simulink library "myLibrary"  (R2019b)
settings: Solver=VariableStepAuto  StartTime=0.0  StopTime=10.0  RelTol=1e-3
undefined symbols (not defined in the file or in its folder): batt_delay, Calculation, cap_1ph, cap_3ph, Complex, Current, Dynamic, EV, ev_charger, EV_ID, ev_num, gcbh, Iabc, Load, max_charge_1ph, max_charge_3ph, max_disch_1ph, max_disch_3ph, MV_LV_transf, myLibrary, phase, Phase, Phasor, rated_1ph, rated_3ph, Single, SoC_init, SPDL, sps_rtmsupport, Tr_capacity, Tstep, Vabc, Vnom, yes
libraries: powerlib x163, $bdroot x13, spsVIMeasurementModel x3, simulink x2, powerlib_meascontrol x1
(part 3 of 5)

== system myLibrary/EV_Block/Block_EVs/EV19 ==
  Breaker : powerlib/Elements/Breaker  InitialState=1  SwitchingTimes=0  External=off  BreakerResistance=0.01  SnubberResistance=1e3  SnubberCapacitance=inf  Measurements=None  MoreParameters=on  NoBreakLoop=off
  Controlled Current Source : powerlib/Electrical Sources/Controlled Current Source  Initialize=on  Source_Type=AC  Amplitude=0  Phase=0  Frequency=50  Measurements=None
  Current Calculation : Subsystem
  Gain : Gain  Gain=sqrt(2)
  Initialization : Subsystem
  Snubber4 : powerlib/Elements/Series RLC Branch  LConnTagsString=__new0  RConnTagsString=__new0  BranchType=R  Resistance=1e6  Inductance=1e-3  SetiL0=off  InitialCurrent=0  Capacitance=1e-6  Setx0=off  InitialVoltage=0  Measurements=None
  Step : Step  Time=0.001  Before=-1  SampleTime=0
  Switch : Switch  Criteria=u2 > Threshold
  Voltage Measurement : powerlib/Measurements/Voltage Measurement  PhasorSimulation=off  OutputType=Complex  PSBequivalent=0
  Phase : PMIOPort  Side=Left
  Neutral : PMIOPort  Port=2  Side=Left
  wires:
  Gain/1 -> Switch/3
  Step/1 -> Switch/2
  Initialization/1(Out1) -> Gain/1
  [Vm_c] -> Switch/1
  [Icontrol] -> Controlled Current Source/1
  Current Calculation/1(Isignal) -> [Icontrol]
  Switch/1 -> Current Calculation/1(Vp)
  Voltage Measurement/1 -> [Vm_c]
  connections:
  Snubber4/LConn1 -- Breaker/LConn1
  Phase/RConn1 -- Voltage Measurement/LConn1 -- Breaker/RConn1 -- Controlled Current Source/LConn1
  Neutral/RConn1 -- Controlled Current Source/RConn1 -- Snubber4/RConn1 -- Voltage Measurement/LConn2

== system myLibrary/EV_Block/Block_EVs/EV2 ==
  Breaker : powerlib/Elements/Breaker  InitialState=1  SwitchingTimes=0  External=off  BreakerResistance=0.01  SnubberResistance=1e3  SnubberCapacitance=inf  Measurements=None  MoreParameters=on  NoBreakLoop=off
  Controlled Current Source : powerlib/Electrical Sources/Controlled Current Source  Initialize=on  Source_Type=AC  Amplitude=0  Phase=0  Frequency=50  Measurements=None
  Current Calculation : Subsystem
  Gain : Gain  Gain=sqrt(2)
  Initialization : Subsystem
  Snubber4 : powerlib/Elements/Series RLC Branch  LConnTagsString=__new0  RConnTagsString=__new0  BranchType=R  Resistance=1e6  Inductance=1e-3  SetiL0=off  InitialCurrent=0  Capacitance=1e-6  Setx0=off  InitialVoltage=0  Measurements=None
  Step : Step  Time=0.001  Before=-1  SampleTime=0
  Switch : Switch  Criteria=u2 > Threshold
  Voltage Measurement : powerlib/Measurements/Voltage Measurement  PhasorSimulation=off  OutputType=Complex  PSBequivalent=0
  Phase : PMIOPort  Side=Left
  Neutral : PMIOPort  Port=2  Side=Left
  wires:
  Gain/1 -> Switch/3
  Step/1 -> Switch/2
  Initialization/1(Out1) -> Gain/1
  [Vm_c] -> Switch/1
  [Icontrol] -> Controlled Current Source/1
  Current Calculation/1(Isignal) -> [Icontrol]
  Switch/1 -> Current Calculation/1(Vp)
  Voltage Measurement/1 -> [Vm_c]
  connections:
  Snubber4/LConn1 -- Breaker/LConn1
  Phase/RConn1 -- Voltage Measurement/LConn1 -- Breaker/RConn1 -- Controlled Current Source/LConn1
  Neutral/RConn1 -- Controlled Current Source/RConn1 -- Snubber4/RConn1 -- Voltage Measurement/LConn2

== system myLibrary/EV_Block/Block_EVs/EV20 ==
  Breaker : powerlib/Elements/Breaker  InitialState=1  SwitchingTimes=0  External=off  BreakerResistance=0.01  SnubberResistance=1e3  SnubberCapacitance=inf  Measurements=None  MoreParameters=on  NoBreakLoop=off
  Controlled Current Source : powerlib/Electrical Sources/Controlled Current Source  Initialize=on  Source_Type=AC  Amplitude=0  Phase=0  Frequency=50  Measurements=None
  Current Calculation : Subsystem
  Gain : Gain  Gain=sqrt(2)
  Initialization : Subsystem
  Snubber4 : powerlib/Elements/Series RLC Branch  LConnTagsString=__new0  RConnTagsString=__new0  BranchType=R  Resistance=1e6  Inductance=1e-3  SetiL0=off  InitialCurrent=0  Capacitance=1e-6  Setx0=off  InitialVoltage=0  Measurements=None
  Step : Step  Time=0.001  Before=-1  SampleTime=0
  Switch : Switch  Criteria=u2 > Threshold
  Voltage Measurement : powerlib/Measurements/Voltage Measurement  PhasorSimulation=off  OutputType=Complex  PSBequivalent=0
  Phase : PMIOPort  Side=Left
  Neutral : PMIOPort  Port=2  Side=Left
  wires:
  Gain/1 -> Switch/3
  Step/1 -> Switch/2
  Initialization/1(Out1) -> Gain/1
  [Vm_c] -> Switch/1
  [Icontrol] -> Controlled Current Source/1
  Current Calculation/1(Isignal) -> [Icontrol]
  Switch/1 -> Current Calculation/1(Vp)
  Voltage Measurement/1 -> [Vm_c]
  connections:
  Snubber4/LConn1 -- Breaker/LConn1
  Phase/RConn1 -- Voltage Measurement/LConn1 -- Breaker/RConn1 -- Controlled Current Source/LConn1
  Neutral/RConn1 -- Controlled Current Source/RConn1 -- Snubber4/RConn1 -- Voltage Measurement/LConn2

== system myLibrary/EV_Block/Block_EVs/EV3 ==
  Breaker : powerlib/Elements/Breaker  InitialState=1  SwitchingTimes=0  External=off  BreakerResistance=0.01  SnubberResistance=1e3  SnubberCapacitance=inf  Measurements=None  MoreParameters=on  NoBreakLoop=off
  Controlled Current Source : powerlib/Electrical Sources/Controlled Current Source  Initialize=on  Source_Type=AC  Amplitude=0  Phase=0  Frequency=50  Measurements=None
  Current Calculation : Subsystem
  Gain : Gain  Gain=sqrt(2)
  Initialization : Subsystem
  Snubber4 : powerlib/Elements/Series RLC Branch  LConnTagsString=__new0  RConnTagsString=__new0  BranchType=R  Resistance=1e6  Inductance=1e-3  SetiL0=off  InitialCurrent=0  Capacitance=1e-6  Setx0=off  InitialVoltage=0  Measurements=None
  Step : Step  Time=0.001  Before=-1  SampleTime=0
  Switch : Switch  Criteria=u2 > Threshold
  Voltage Measurement : powerlib/Measurements/Voltage Measurement  PhasorSimulation=off  OutputType=Complex  PSBequivalent=0
  Phase : PMIOPort  Side=Left
  Neutral : PMIOPort  Port=2  Side=Left
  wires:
  Gain/1 -> Switch/3
  Step/1 -> Switch/2
  Initialization/1(Out1) -> Gain/1
  [Vm_c] -> Switch/1
  [Icontrol] -> Controlled Current Source/1
  Current Calculation/1(Isignal) -> [Icontrol]
  Switch/1 -> Current Calculation/1(Vp)
  Voltage Measurement/1 -> [Vm_c]
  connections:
  Snubber4/LConn1 -- Breaker/LConn1
  Phase/RConn1 -- Voltage Measurement/LConn1 -- Breaker/RConn1 -- Controlled Current Source/LConn1
  Neutral/RConn1 -- Controlled Current Source/RConn1 -- Snubber4/RConn1 -- Voltage Measurement/LConn2

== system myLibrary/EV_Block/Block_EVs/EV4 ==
  Breaker : powerlib/Elements/Breaker  InitialState=1  SwitchingTimes=0  External=off  BreakerResistance=0.01  SnubberResistance=1e3  SnubberCapacitance=inf  Measurements=None  MoreParameters=on  NoBreakLoop=off
  Controlled Current Source : powerlib/Electrical Sources/Controlled Current Source  Initialize=on  Source_Type=AC  Amplitude=0  Phase=0  Frequency=50  Measurements=None
  Current Calculation : Subsystem
  Gain : Gain  Gain=sqrt(2)
  Initialization : Subsystem
  Snubber4 : powerlib/Elements/Series RLC Branch  LConnTagsString=__new0  RConnTagsString=__new0  BranchType=R  Resistance=1e6  Inductance=1e-3  SetiL0=off  InitialCurrent=0  Capacitance=1e-6  Setx0=off  InitialVoltage=0  Measurements=None
  Step : Step  Time=0.001  Before=-1  SampleTime=0
  Switch : Switch  Criteria=u2 > Threshold
  Voltage Measurement : powerlib/Measurements/Voltage Measurement  PhasorSimulation=off  OutputType=Complex  PSBequivalent=0
  Phase : PMIOPort  Side=Left
  Neutral : PMIOPort  Port=2  Side=Left
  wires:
  Gain/1 -> Switch/3
  Step/1 -> Switch/2
  Initialization/1(Out1) -> Gain/1
  [Vm_c] -> Switch/1
  [Icontrol] -> Controlled Current Source/1
  Current Calculation/1(Isignal) -> [Icontrol]
  Switch/1 -> Current Calculation/1(Vp)
  Voltage Measurement/1 -> [Vm_c]
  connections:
  Snubber4/LConn1 -- Breaker/LConn1
  Phase/RConn1 -- Voltage Measurement/LConn1 -- Breaker/RConn1 -- Controlled Current Source/LConn1
  Neutral/RConn1 -- Controlled Current Source/RConn1 -- Snubber4/RConn1 -- Voltage Measurement/LConn2

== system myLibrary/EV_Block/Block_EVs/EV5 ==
  Breaker : powerlib/Elements/Breaker  InitialState=1  SwitchingTimes=0  External=off  BreakerResistance=0.01  SnubberResistance=1e3  SnubberCapacitance=inf  Measurements=None  MoreParameters=on  NoBreakLoop=off
  Controlled Current Source : powerlib/Electrical Sources/Controlled Current Source  Initialize=on  Source_Type=AC  Amplitude=0  Phase=0  Frequency=50  Measurements=None
  Current Calculation : Subsystem
  Gain : Gain  Gain=sqrt(2)
  Initialization : Subsystem
  Snubber4 : powerlib/Elements/Series RLC Branch  LConnTagsString=__new0  RConnTagsString=__new0  BranchType=R  Resistance=1e6  Inductance=1e-3  SetiL0=off  InitialCurrent=0  Capacitance=1e-6  Setx0=off  InitialVoltage=0  Measurements=None
  Step : Step  Time=0.001  Before=-1  SampleTime=0
  Switch : Switch  Criteria=u2 > Threshold
  Voltage Measurement : powerlib/Measurements/Voltage Measurement  PhasorSimulation=off  OutputType=Complex  PSBequivalent=0
  Phase : PMIOPort  Side=Left
  Neutral : PMIOPort  Port=2  Side=Left
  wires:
  Gain/1 -> Switch/3
  Step/1 -> Switch/2
  Initialization/1(Out1) -> Gain/1
  [Vm_c] -> Switch/1
  [Icontrol] -> Controlled Current Source/1
  Current Calculation/1(Isignal) -> [Icontrol]
  Switch/1 -> Current Calculation/1(Vp)
  Voltage Measurement/1 -> [Vm_c]
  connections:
  Snubber4/LConn1 -- Breaker/LConn1
  Phase/RConn1 -- Voltage Measurement/LConn1 -- Breaker/RConn1 -- Controlled Current Source/LConn1
  Neutral/RConn1 -- Controlled Current Source/RConn1 -- Snubber4/RConn1 -- Voltage Measurement/LConn2

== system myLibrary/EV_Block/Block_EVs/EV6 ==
  Breaker : powerlib/Elements/Breaker  InitialState=1  SwitchingTimes=0  External=off  BreakerResistance=0.01  SnubberResistance=1e3  SnubberCapacitance=inf  Measurements=None  MoreParameters=on  NoBreakLoop=off
  Controlled Current Source : powerlib/Electrical Sources/Controlled Current Source  Initialize=on  Source_Type=AC  Amplitude=0  Phase=0  Frequency=50  Measurements=None
  Current Calculation : Subsystem
  Gain : Gain  Gain=sqrt(2)
  Initialization : Subsystem
  Snubber4 : powerlib/Elements/Series RLC Branch  LConnTagsString=__new0  RConnTagsString=__new0  BranchType=R  Resistance=1e6  Inductance=1e-3  SetiL0=off  InitialCurrent=0  Capacitance=1e-6  Setx0=off  InitialVoltage=0  Measurements=None
  Step : Step  Time=0.001  Before=-1  SampleTime=0
  Switch : Switch  Criteria=u2 > Threshold
  Voltage Measurement : powerlib/Measurements/Voltage Measurement  PhasorSimulation=off  OutputType=Complex  PSBequivalent=0
  Phase : PMIOPort  Side=Left
  Neutral : PMIOPort  Port=2  Side=Left
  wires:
  Gain/1 -> Switch/3
  Step/1 -> Switch/2
  Initialization/1(Out1) -> Gain/1
  [Vm_c] -> Switch/1
  [Icontrol] -> Controlled Current Source/1
  Current Calculation/1(Isignal) -> [Icontrol]
  Switch/1 -> Current Calculation/1(Vp)
  Voltage Measurement/1 -> [Vm_c]
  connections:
  Snubber4/LConn1 -- Breaker/LConn1
  Phase/RConn1 -- Voltage Measurement/LConn1 -- Breaker/RConn1 -- Controlled Current Source/LConn1
  Neutral/RConn1 -- Controlled Current Source/RConn1 -- Snubber4/RConn1 -- Voltage Measurement/LConn2

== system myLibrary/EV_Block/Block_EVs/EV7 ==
  Breaker : powerlib/Elements/Breaker  InitialState=1  SwitchingTimes=0  External=off  BreakerResistance=0.01  SnubberResistance=1e3  SnubberCapacitance=inf  Measurements=None  MoreParameters=on  NoBreakLoop=off
  Controlled Current Source : powerlib/Electrical Sources/Controlled Current Source  Initialize=on  Source_Type=AC  Amplitude=0  Phase=0  Frequency=50  Measurements=None
  Current Calculation : Subsystem
  Gain : Gain  Gain=sqrt(2)
  Initialization : Subsystem
  Snubber4 : powerlib/Elements/Series RLC Branch  LConnTagsString=__new0  RConnTagsString=__new0  BranchType=R  Resistance=1e6  Inductance=1e-3  SetiL0=off  InitialCurrent=0  Capacitance=1e-6  Setx0=off  InitialVoltage=0  Measurements=None
  Step : Step  Time=0.001  Before=-1  SampleTime=0
  Switch : Switch  Criteria=u2 > Threshold
  Voltage Measurement : powerlib/Measurements/Voltage Measurement  PhasorSimulation=off  OutputType=Complex  PSBequivalent=0
  Phase : PMIOPort  Side=Left
  Neutral : PMIOPort  Port=2  Side=Left
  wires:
  Gain/1 -> Switch/3
  Step/1 -> Switch/2
  Initialization/1(Out1) -> Gain/1
  [Vm_c] -> Switch/1
  [Icontrol] -> Controlled Current Source/1
  Current Calculation/1(Isignal) -> [Icontrol]
  Switch/1 -> Current Calculation/1(Vp)
  Voltage Measurement/1 -> [Vm_c]
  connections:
  Snubber4/LConn1 -- Breaker/LConn1
  Phase/RConn1 -- Voltage Measurement/LConn1 -- Breaker/RConn1 -- Controlled Current Source/LConn1
  Neutral/RConn1 -- Controlled Current Source/RConn1 -- Snubber4/RConn1 -- Voltage Measurement/LConn2

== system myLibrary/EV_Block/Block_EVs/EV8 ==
  Breaker : powerlib/Elements/Breaker  InitialState=1  SwitchingTimes=0  External=off  BreakerResistance=0.01  SnubberResistance=1e3  SnubberCapacitance=inf  Measurements=None  MoreParameters=on  NoBreakLoop=off
  Controlled Current Source : powerlib/Electrical Sources/Controlled Current Source  Initialize=on  Source_Type=AC  Amplitude=0  Phase=0  Frequency=50  Measurements=None
  Current Calculation : Subsystem
  Gain : Gain  Gain=sqrt(2)
  Initialization : Subsystem
  Snubber4 : powerlib/Elements/Series RLC Branch  LConnTagsString=__new0  RConnTagsString=__new0  BranchType=R  Resistance=1e6  Inductance=1e-3  SetiL0=off  InitialCurrent=0  Capacitance=1e-6  Setx0=off  InitialVoltage=0  Measurements=None
  Step : Step  Time=0.001  Before=-1  SampleTime=0
  Switch : Switch  Criteria=u2 > Threshold
  Voltage Measurement : powerlib/Measurements/Voltage Measurement  PhasorSimulation=off  OutputType=Complex  PSBequivalent=0
  Phase : PMIOPort  Side=Left
  Neutral : PMIOPort  Port=2  Side=Left
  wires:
  Gain/1 -> Switch/3
  Step/1 -> Switch/2
  Initialization/1(Out1) -> Gain/1
  [Vm_c] -> Switch/1
  [Icontrol] -> Controlled Current Source/1
  Current Calculation/1(Isignal) -> [Icontrol]
  Switch/1 -> Current Calculation/1(Vp)
  Voltage Measurement/1 -> [Vm_c]
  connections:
  Snubber4/LConn1 -- Breaker/LConn1
  Phase/RConn1 -- Voltage Measurement/LConn1 -- Breaker/RConn1 -- Controlled Current Source/LConn1
  Neutral/RConn1 -- Controlled Current Source/RConn1 -- Snubber4/RConn1 -- Voltage Measurement/LConn2

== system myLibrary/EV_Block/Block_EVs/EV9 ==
  Breaker : powerlib/Elements/Breaker  InitialState=1  SwitchingTimes=0  External=off  BreakerResistance=0.01  SnubberResistance=1e3  SnubberCapacitance=inf  Measurements=None  MoreParameters=on  NoBreakLoop=off
  Controlled Current Source : powerlib/Electrical Sources/Controlled Current Source  Initialize=on  Source_Type=AC  Amplitude=0  Phase=0  Frequency=50  Measurements=None
  Current Calculation : Subsystem
  Gain : Gain  Gain=sqrt(2)
  Initialization : Subsystem
  Snubber4 : powerlib/Elements/Series RLC Branch  LConnTagsString=__new0  RConnTagsString=__new0  BranchType=R  Resistance=1e6  Inductance=1e-3  SetiL0=off  InitialCurrent=0  Capacitance=1e-6  Setx0=off  InitialVoltage=0  Measurements=None
  Step : Step  Time=0.001  Before=-1  SampleTime=0
  Switch : Switch  Criteria=u2 > Threshold
  Voltage Measurement : powerlib/Measurements/Voltage Measurement  PhasorSimulation=off  OutputType=Complex  PSBequivalent=0
  Phase : PMIOPort  Side=Left
  Neutral : PMIOPort  Port=2  Side=Left
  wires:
  Gain/1 -> Switch/3
  Step/1 -> Switch/2
  Initialization/1(Out1) -> Gain/1
  [Vm_c] -> Switch/1
  [Icontrol] -> Controlled Current Source/1
  Current Calculation/1(Isignal) -> [Icontrol]
  Switch/1 -> Current Calculation/1(Vp)
  Voltage Measurement/1 -> [Vm_c]
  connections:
  Snubber4/LConn1 -- Breaker/LConn1
  Phase/RConn1 -- Voltage Measurement/LConn1 -- Breaker/RConn1 -- Controlled Current Source/LConn1
  Neutral/RConn1 -- Controlled Current Source/RConn1 -- Snubber4/RConn1 -- Voltage Measurement/LConn2

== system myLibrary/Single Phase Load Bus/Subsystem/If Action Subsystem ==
  Action Port : ActionPort
  Constant : Constant
  Out1 : Outport  VectorParamsAs1DForOutWhenUnconnected=off
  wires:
  Constant/1 -> Out1/1

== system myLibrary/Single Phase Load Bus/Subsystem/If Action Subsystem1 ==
  Action Port : ActionPort
  Constant : Constant
  Out1 : Outport  VectorParamsAs1DForOutWhenUnconnected=off
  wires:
  Constant/1 -> Out1/1

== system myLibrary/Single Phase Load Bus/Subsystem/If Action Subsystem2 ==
  Action Port : ActionPort
  Constant : Constant
  Out1 : Outport  VectorParamsAs1DForOutWhenUnconnected=off
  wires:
  Constant/1 -> Out1/1

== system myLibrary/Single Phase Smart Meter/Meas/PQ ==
  V : Inport
  I : Inport  Port=2
  Complex to Real-Imag : ComplexToRealImag
  Constant : Constant  Value=2
  Divide : Product  Inputs=*/
  Math Function : Math  Operator=conj
  Product : Product
  P : Outport  VectorParamsAs1DForOutWhenUnconnected=off
  Q : Outport  Port=2  VectorParamsAs1DForOutWhenUnconnected=off
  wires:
  I/1 -> Math Function/1
  V/1 -> Product/1
  Math Function/1 -> Product/2
  Product/1 -> Divide/1
  Constant/1 -> Divide/2
  Divide/1 -> Complex to Real-Imag/1
  Complex to Real-Imag/1 -> P/1
  Complex to Real-Imag/2 -> Q/1

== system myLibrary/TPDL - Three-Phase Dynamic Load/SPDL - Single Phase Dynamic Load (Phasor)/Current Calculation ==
  Vp : Inport
  Demux : Demux  Outputs=6
  Divide : Product  Inputs=*/
  From Workspace : FromWorkspace  VariableName=Load_Profile  SampleTime=0  OutputAfterFinalValue=Holding final value
  Gain : Gain  Gain=2
  Math Function : Math  Operator=conj
  Real-Imag to Complex : RealImagToComplex
  Isignal : Outport  VectorParamsAs1DForOutWhenUnconnected=off
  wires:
  Vp/1 -> Divide/2
  Gain/1 -> Divide/1
  Divide/1 -> Math Function/1
  Math Function/1 -> Isignal/1
  From Workspace/1 -> Demux/1
  Demux/1 -> Real-Imag to Complex/1
  Demux/2 -> Real-Imag to Complex/2
  Real-Imag to Complex/1 -> Gain/1

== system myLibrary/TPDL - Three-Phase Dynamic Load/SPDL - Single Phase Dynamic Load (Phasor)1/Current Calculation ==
  Vp : Inport
  Demux : Demux  Outputs=6
  Divide : Product  Inputs=*/
  From Workspace : FromWorkspace  VariableName=Load_Profile  SampleTime=0  OutputAfterFinalValue=Holding final value
  Gain : Gain  Gain=2
  Math Function : Math  Operator=conj
  Real-Imag to Complex : RealImagToComplex
  Isignal : Outport  VectorParamsAs1DForOutWhenUnconnected=off
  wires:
  Vp/1 -> Divide/2
  Gain/1 -> Divide/1
  Divide/1 -> Math Function/1
  Math Function/1 -> Isignal/1
  From Workspace/1 -> Demux/1
  Demux/3 -> Real-Imag to Complex/1
  Demux/4 -> Real-Imag to Complex/2
  Real-Imag to Complex/1 -> Gain/1

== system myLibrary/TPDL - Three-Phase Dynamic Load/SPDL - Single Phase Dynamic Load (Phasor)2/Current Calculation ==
  Vp : Inport
  Demux : Demux  Outputs=6
  Divide : Product  Inputs=*/
  From Workspace : FromWorkspace  VariableName=Load_Profile  SampleTime=0  OutputAfterFinalValue=Holding final value
  Gain : Gain  Gain=2
  Math Function : Math  Operator=conj
  Real-Imag to Complex : RealImagToComplex
  Isignal : Outport  VectorParamsAs1DForOutWhenUnconnected=off
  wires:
  Vp/1 -> Divide/2
  Gain/1 -> Divide/1
  Divide/1 -> Math Function/1
  Math Function/1 -> Isignal/1
  From Workspace/1 -> Demux/1
  Demux/5 -> Real-Imag to Complex/1
  Demux/6 -> Real-Imag to Complex/2
  Real-Imag to Complex/1 -> Gain/1

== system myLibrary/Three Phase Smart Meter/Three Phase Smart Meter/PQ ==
  V : Inport
  I : Inport  Port=2
  Complex to Real-Imag : ComplexToRealImag
  Constant : Constant  Value=2
  Divide : Product  Inputs=*/
  Math Function : Math  Operator=conj
  Product : Product
  P : Outport  VectorParamsAs1DForOutWhenUnconnected=off
  Q : Outport  Port=2  VectorParamsAs1DForOutWhenUnconnected=off
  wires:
  I/1 -> Math Function/1
  V/1 -> Product/1
  Math Function/1 -> Product/2
  Product/1 -> Divide/1
  Constant/1 -> Divide/2
  Divide/1 -> Complex to Real-Imag/1
  Complex to Real-Imag/1 -> P/1
  Complex to Real-Imag/2 -> Q/1

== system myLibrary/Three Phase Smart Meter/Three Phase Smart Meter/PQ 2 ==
  V : Inport
  I : Inport  Port=2
  Complex to Real-Imag : ComplexToRealImag
  Constant : Constant  Value=2
  Divide : Product  Inputs=*/
  Math Function : Math  Operator=conj
  Product : Product
  P : Outport  VectorParamsAs1DForOutWhenUnconnected=off
  Q : Outport  Port=2  VectorParamsAs1DForOutWhenUnconnected=off
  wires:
  I/1 -> Math Function/1
  V/1 -> Product/1
  Math Function/1 -> Product/2
  Product/1 -> Divide/1
  Constant/1 -> Divide/2
  Divide/1 -> Complex to Real-Imag/1
  Complex to Real-Imag/1 -> P/1
  Complex to Real-Imag/2 -> Q/1

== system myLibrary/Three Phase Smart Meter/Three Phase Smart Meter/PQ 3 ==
  V : Inport
  I : Inport  Port=2
  Complex to Real-Imag : ComplexToRealImag
  Constant : Constant  Value=2
  Divide : Product  Inputs=*/
  Math Function : Math  Operator=conj
  Product : Product
  P : Outport  VectorParamsAs1DForOutWhenUnconnected=off
  Q : Outport  Port=2  VectorParamsAs1DForOutWhenUnconnected=off
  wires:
  I/1 -> Math Function/1
  V/1 -> Product/1
  Math Function/1 -> Product/2
  Product/1 -> Divide/1
  Constant/1 -> Divide/2
  Divide/1 -> Complex to Real-Imag/1
  Complex to Real-Imag/1 -> P/1
  Complex to Real-Imag/2 -> Q/1

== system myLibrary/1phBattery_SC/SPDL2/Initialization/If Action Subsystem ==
  Action Port : ActionPort
  Constant : Constant
  Out1 : Outport  VectorParamsAs1DForOutWhenUnconnected=off
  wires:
  Constant/1 -> Out1/1

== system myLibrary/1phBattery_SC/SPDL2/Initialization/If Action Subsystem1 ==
  Action Port : ActionPort
  Constant : Constant
  Out1 : Outport  VectorParamsAs1DForOutWhenUnconnected=off
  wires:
  Constant/1 -> Out1/1

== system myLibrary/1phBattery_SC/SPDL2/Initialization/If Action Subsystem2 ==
  Action Port : ActionPort
  Constant : Constant
  Out1 : Outport  VectorParamsAs1DForOutWhenUnconnected=off
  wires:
  Constant/1 -> Out1/1

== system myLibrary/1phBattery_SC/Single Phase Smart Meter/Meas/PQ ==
  V : Inport
  I : Inport  Port=2
  Complex to Real-Imag : ComplexToRealImag
  Constant : Constant  Value=2
  Divide : Product  Inputs=*/
  Math Function : Math  Operator=conj
  Product : Product
  P : Outport  VectorParamsAs1DForOutWhenUnconnected=off
  Q : Outport  Port=2  VectorParamsAs1DForOutWhenUnconnected=off
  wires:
  Complex to Real-Imag/2 -> Q/1
  Complex to Real-Imag/1 -> P/1
  Divide/1 -> Complex to Real-Imag/1
  Constant/1 -> Divide/2
  Product/1 -> Divide/1
  Math Function/1 -> Product/2
  V/1 -> Product/1
  I/1 -> Math Function/1

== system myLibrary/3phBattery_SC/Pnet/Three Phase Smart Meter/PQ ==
  V : Inport
  I : Inport  Port=2
  Complex to Real-Imag : ComplexToRealImag
  Constant : Constant  Value=2
  Divide : Product  Inputs=*/
  Math Function : Math  Operator=conj
  Product : Product
  P : Outport  VectorParamsAs1DForOutWhenUnconnected=off
  Q : Outport  Port=2  VectorParamsAs1DForOutWhenUnconnected=off
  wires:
  I/1 -> Math Function/1
  V/1 -> Product/1
  Math Function/1 -> Product/2
  Product/1 -> Divide/1
  Constant/1 -> Divide/2
  Divide/1 -> Complex to Real-Imag/1
  Complex to Real-Imag/1 -> P/1
  Complex to Real-Imag/2 -> Q/1

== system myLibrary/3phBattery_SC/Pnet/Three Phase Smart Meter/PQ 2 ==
  V : Inport
  I : Inport  Port=2
  Complex to Real-Imag : ComplexToRealImag
  Constant : Constant  Value=2
  Divide : Product  Inputs=*/
  Math Function : Math  Operator=conj
  Product : Product
  P : Outport  VectorParamsAs1DForOutWhenUnconnected=off
  Q : Outport  Port=2  VectorParamsAs1DForOutWhenUnconnected=off
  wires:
  I/1 -> Math Function/1
  V/1 -> Product/1
  Math Function/1 -> Product/2
  Product/1 -> Divide/1
  Constant/1 -> Divide/2
  Divide/1 -> Complex to Real-Imag/1
  Complex to Real-Imag/1 -> P/1
  Complex to Real-Imag/2 -> Q/1

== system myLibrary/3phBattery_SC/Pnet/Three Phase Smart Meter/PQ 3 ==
  V : Inport
  I : Inport  Port=2
  Complex to Real-Imag : ComplexToRealImag
  Constant : Constant  Value=2
  Divide : Product  Inputs=*/
  Math Function : Math  Operator=conj
  Product : Product
  P : Outport  VectorParamsAs1DForOutWhenUnconnected=off
  Q : Outport  Port=2  VectorParamsAs1DForOutWhenUnconnected=off
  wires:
  I/1 -> Math Function/1
  V/1 -> Product/1
  Math Function/1 -> Product/2
  Product/1 -> Divide/1
  Constant/1 -> Divide/2
  Divide/1 -> Complex to Real-Imag/1
  Complex to Real-Imag/1 -> P/1
  Complex to Real-Imag/2 -> Q/1

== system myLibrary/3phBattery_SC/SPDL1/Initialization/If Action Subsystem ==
  Action Port : ActionPort
  Constant : Constant
  Out1 : Outport  VectorParamsAs1DForOutWhenUnconnected=off
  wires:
  Constant/1 -> Out1/1

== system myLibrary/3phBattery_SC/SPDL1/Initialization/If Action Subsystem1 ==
  Action Port : ActionPort
  Constant : Constant
  Out1 : Outport  VectorParamsAs1DForOutWhenUnconnected=off
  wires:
  Constant/1 -> Out1/1

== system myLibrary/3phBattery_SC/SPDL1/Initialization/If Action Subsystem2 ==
  Action Port : ActionPort
  Constant : Constant
  Out1 : Outport  VectorParamsAs1DForOutWhenUnconnected=off
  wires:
  Constant/1 -> Out1/1

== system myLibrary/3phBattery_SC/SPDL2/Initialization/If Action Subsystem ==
  Action Port : ActionPort
  Constant : Constant
  Out1 : Outport  VectorParamsAs1DForOutWhenUnconnected=off
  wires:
  Constant/1 -> Out1/1

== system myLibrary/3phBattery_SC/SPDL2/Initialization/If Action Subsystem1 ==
  Action Port : ActionPort
  Constant : Constant
  Out1 : Outport  VectorParamsAs1DForOutWhenUnconnected=off
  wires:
  Constant/1 -> Out1/1

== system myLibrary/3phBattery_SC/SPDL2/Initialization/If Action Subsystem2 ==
  Action Port : ActionPort
  Constant : Constant
  Out1 : Outport  VectorParamsAs1DForOutWhenUnconnected=off
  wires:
  Constant/1 -> Out1/1

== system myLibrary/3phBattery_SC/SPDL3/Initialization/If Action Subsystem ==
  Action Port : ActionPort
  Constant : Constant
  Out1 : Outport  VectorParamsAs1DForOutWhenUnconnected=off
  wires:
  Constant/1 -> Out1/1

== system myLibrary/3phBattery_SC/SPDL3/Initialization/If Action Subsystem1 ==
  Action Port : ActionPort
  Constant : Constant
  Out1 : Outport  VectorParamsAs1DForOutWhenUnconnected=off
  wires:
  Constant/1 -> Out1/1

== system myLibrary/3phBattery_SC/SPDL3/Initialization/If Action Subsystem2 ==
  Action Port : ActionPort
  Constant : Constant
  Out1 : Outport  VectorParamsAs1DForOutWhenUnconnected=off
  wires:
  Constant/1 -> Out1/1

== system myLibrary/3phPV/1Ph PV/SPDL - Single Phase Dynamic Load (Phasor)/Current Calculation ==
  Vp : Inport
  From Workspace : FromWorkspace  VariableName=Load_Profile  SampleTime=0  OutputAfterFinalValue=Holding final value
  Q_V : Subsystem  Commented=on  mask{pf_V=0.9, Vpoints=[0.9 0.97 1.03 1.1]}
  constant pf : Subsystem  mask{pf=0.9}
  cosf_(P,V) : Subsystem  Commented=on  mask{Pstart=0.4, pfend=0.9, Vstart=1.03}
      mask prompts: Vstart "Vstart [pu]"
  cosf_P : Subsystem  Commented=on  mask{Pstart=0.4, pfend=0.9}
  dynamic curtailment : Subsystem  Commented=on  mask{Pmin=0, Vstart=1.08, Vend=1.12}
      mask prompts: Pmin "Pmin [pu]"; Vstart "Vstart [pu]"; Vend "Vend [pu]"
  fix Q : Subsystem  Commented=on  mask{pf=0.9}
      mask prompts: pf "pf (Q is calculated as Q=Pcapacity*tan(theta))"
  static curtailment : Saturate  UpperLimit=1  LowerLimit=0
  Isignal : Outport  VectorParamsAs1DForOutWhenUnconnected=off
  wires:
  Vp/1 -> dynamic curtailment/1(Vp), Q_V/1(Vp), cosf_(P,V)/1(Vp), fix Q/1(Vp), cosf_P/1(Vp), constant pf/1(Vp)
  static curtailment/1 -> constant pf/2(LP), Q_V/2(LP), cosf_(P,V)/2(LP), fix Q/2(LP), cosf_P/2(LP)
  constant pf/1(Isignal) -> Isignal/1
  From Workspace/1 -> static curtailment/1

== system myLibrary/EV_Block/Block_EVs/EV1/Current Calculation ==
  Vp : Inport
  Constant : Constant  Commented=on  Value=2060
  Constant1 : Constant  Commented=on  Value=600
  Demux : Demux  Outputs=2
  Divide : Product  Inputs=*/
  From Workspace : FromWorkspace  VariableName=Load_Profile  SampleTime=0  OutputAfterFinalValue=Holding final value
  Gain : Gain  Gain=2
  Math Function : Math  Operator=conj
  Real-Imag to Complex : RealImagToComplex
  Isignal : Outport  VectorParamsAs1DForOutWhenUnconnected=off
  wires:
  Demux/2 -> Real-Imag to Complex/2
  Demux/1 -> Real-Imag to Complex/1
  Math Function/1 -> Isignal/1
  Divide/1 -> Math Function/1
  Gain/1 -> Divide/1
  Vp/1 -> Divide/2
  Real-Imag to Complex/1 -> Gain/1
  From Workspace/1 -> Demux/1

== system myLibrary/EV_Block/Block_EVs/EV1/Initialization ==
  Constant : Constant  Value=207.85
  Constant1 : Constant  Value=-120
  Constant2 : Constant  Value=-207.85
  Constant3 : Constant  Value=-120
  Constant4 : Constant  Value=0
  Constant5 : Constant  Value=240
  Constant6 : Constant  Value=Phase
  Data Type Conversion : DataTypeConversion  OutDataTypeStr=double
  Demux : Demux  Outputs=2
  If : If  IfExpression=u1 == 1  ElseIfExpressions=u1 == 2
  If Action Subsystem : Subsystem  TreatAsAtomicUnit=on
  If Action Subsystem1 : Subsystem  TreatAsAtomicUnit=on
  If Action Subsystem2 : Subsystem  TreatAsAtomicUnit=on
  Logical Operator : Logic  Operator=NOT  AllPortsSameDT=off  OutDataTypeStr=boolean
  Mux : Mux  Inputs=2
  Real-Imag to Complex : RealImagToComplex
  Real-Imag to Complex1 : RealImagToComplex
  Real-Imag to Complex2 : RealImagToComplex
  Switch : Switch  Criteria=u2 > Threshold
  Switch1 : Switch  Criteria=u2 > Threshold
  Out1 : Outport  VectorParamsAs1DForOutWhenUnconnected=off
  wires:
  Data Type Conversion/1 -> Mux/2
  [control] -> Demux/1
  Logical Operator/1 -> Data Type Conversion/1
  If Action Subsystem/1(Out1) -> Mux/1
  Mux/1 -> [control]
  If Action Subsystem2/1(Out1) -> Logical Operator/1
  Demux/2 -> Switch1/2
  Demux/1 -> Switch/2
  If/3 -> If Action Subsystem2/Action
  If/2 -> If Action Subsystem1/Action
  If/1 -> If Action Subsystem/Action
  Constant6/1 -> If/1
  Switch1/1 -> Out1/1
  Real-Imag to Complex2/1 -> Switch1/3
  Switch/1 -> Switch1/1
  Real-Imag to Complex1/1 -> Switch/3
  Real-Imag to Complex/1 -> Switch/1
  Constant4/1 -> Real-Imag to Complex2/1
  Constant5/1 -> Real-Imag to Complex2/2
  Constant2/1 -> Real-Imag to Complex1/1
  Constant3/1 -> Real-Imag to Complex1/2
  Constant/1 -> Real-Imag to Complex/1
  Constant1/1 -> Real-Imag to Complex/2

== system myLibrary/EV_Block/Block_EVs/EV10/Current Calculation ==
  Vp : Inport
  Constant : Constant  Commented=on  Value=2060
  Constant1 : Constant  Commented=on  Value=600
  Demux : Demux  Outputs=2
  Divide : Product  Inputs=*/
  From Workspace : FromWorkspace  VariableName=Load_Profile  SampleTime=0  OutputAfterFinalValue=Holding final value
  Gain : Gain  Gain=2
  Math Function : Math  Operator=conj
  Real-Imag to Complex : RealImagToComplex
  Isignal : Outport  VectorParamsAs1DForOutWhenUnconnected=off
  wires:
  Demux/2 -> Real-Imag to Complex/2
  Demux/1 -> Real-Imag to Complex/1
  Math Function/1 -> Isignal/1
  Divide/1 -> Math Function/1
  Gain/1 -> Divide/1
  Vp/1 -> Divide/2
  Real-Imag to Complex/1 -> Gain/1
  From Workspace/1 -> Demux/1

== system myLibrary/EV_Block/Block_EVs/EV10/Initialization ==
  Constant : Constant  Value=207.85
  Constant1 : Constant  Value=-120
  Constant2 : Constant  Value=-207.85
  Constant3 : Constant  Value=-120
  Constant4 : Constant  Value=0
  Constant5 : Constant  Value=240
  Constant6 : Constant  Value=Phase
  Data Type Conversion : DataTypeConversion  OutDataTypeStr=double
  Demux : Demux  Outputs=2
  If : If  IfExpression=u1 == 1  ElseIfExpressions=u1 == 2
  If Action Subsystem : Subsystem  TreatAsAtomicUnit=on
  If Action Subsystem1 : Subsystem  TreatAsAtomicUnit=on
  If Action Subsystem2 : Subsystem  TreatAsAtomicUnit=on
  Logical Operator : Logic  Operator=NOT  AllPortsSameDT=off  OutDataTypeStr=boolean
  Mux : Mux  Inputs=2
  Real-Imag to Complex : RealImagToComplex
  Real-Imag to Complex1 : RealImagToComplex
  Real-Imag to Complex2 : RealImagToComplex
  Switch : Switch  Criteria=u2 > Threshold
  Switch1 : Switch  Criteria=u2 > Threshold
  Out1 : Outport  VectorParamsAs1DForOutWhenUnconnected=off
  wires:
  Data Type Conversion/1 -> Mux/2
  [control] -> Demux/1
  Logical Operator/1 -> Data Type Conversion/1
  If Action Subsystem/1(Out1) -> Mux/1
  Mux/1 -> [control]
  If Action Subsystem2/1(Out1) -> Logical Operator/1
  Demux/2 -> Switch1/2
  Demux/1 -> Switch/2
  If/3 -> If Action Subsystem2/Action
  If/2 -> If Action Subsystem1/Action
  If/1 -> If Action Subsystem/Action
  Constant6/1 -> If/1
  Switch1/1 -> Out1/1
  Real-Imag to Complex2/1 -> Switch1/3
  Switch/1 -> Switch1/1
  Real-Imag to Complex1/1 -> Switch/3
  Real-Imag to Complex/1 -> Switch/1
  Constant4/1 -> Real-Imag to Complex2/1
  Constant5/1 -> Real-Imag to Complex2/2
  Constant2/1 -> Real-Imag to Complex1/1
  Constant3/1 -> Real-Imag to Complex1/2
  Constant/1 -> Real-Imag to Complex/1
  Constant1/1 -> Real-Imag to Complex/2

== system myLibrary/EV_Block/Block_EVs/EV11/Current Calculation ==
  Vp : Inport
  Constant : Constant  Commented=on  Value=2060
  Constant1 : Constant  Commented=on  Value=600
  Demux : Demux  Outputs=2
  Divide : Product  Inputs=*/
  From Workspace : FromWorkspace  VariableName=Load_Profile  SampleTime=0  OutputAfterFinalValue=Holding final value
  Gain : Gain  Gain=2
  Math Function : Math  Operator=conj
  Real-Imag to Complex : RealImagToComplex
  Isignal : Outport  VectorParamsAs1DForOutWhenUnconnected=off
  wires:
  Demux/2 -> Real-Imag to Complex/2
  Demux/1 -> Real-Imag to Complex/1
  Math Function/1 -> Isignal/1
  Divide/1 -> Math Function/1
  Gain/1 -> Divide/1
  Vp/1 -> Divide/2
  Real-Imag to Complex/1 -> Gain/1
  From Workspace/1 -> Demux/1

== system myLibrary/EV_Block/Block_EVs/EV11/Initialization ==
  Constant : Constant  Value=207.85
  Constant1 : Constant  Value=-120
  Constant2 : Constant  Value=-207.85
  Constant3 : Constant  Value=-120
  Constant4 : Constant  Value=0
  Constant5 : Constant  Value=240
  Constant6 : Constant  Value=Phase
  Data Type Conversion : DataTypeConversion  OutDataTypeStr=double
  Demux : Demux  Outputs=2
  If : If  IfExpression=u1 == 1  ElseIfExpressions=u1 == 2
  If Action Subsystem : Subsystem  TreatAsAtomicUnit=on
  If Action Subsystem1 : Subsystem  TreatAsAtomicUnit=on
  If Action Subsystem2 : Subsystem  TreatAsAtomicUnit=on
  Logical Operator : Logic  Operator=NOT  AllPortsSameDT=off  OutDataTypeStr=boolean
  Mux : Mux  Inputs=2
  Real-Imag to Complex : RealImagToComplex
  Real-Imag to Complex1 : RealImagToComplex
  Real-Imag to Complex2 : RealImagToComplex
  Switch : Switch  Criteria=u2 > Threshold
  Switch1 : Switch  Criteria=u2 > Threshold
  Out1 : Outport  VectorParamsAs1DForOutWhenUnconnected=off
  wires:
  Data Type Conversion/1 -> Mux/2
  [control] -> Demux/1
  Logical Operator/1 -> Data Type Conversion/1
  If Action Subsystem/1(Out1) -> Mux/1
  Mux/1 -> [control]
  If Action Subsystem2/1(Out1) -> Logical Operator/1
  Demux/2 -> Switch1/2
  Demux/1 -> Switch/2
  If/3 -> If Action Subsystem2/Action
  If/2 -> If Action Subsystem1/Action
  If/1 -> If Action Subsystem/Action
  Constant6/1 -> If/1
  Switch1/1 -> Out1/1
  Real-Imag to Complex2/1 -> Switch1/3
  Switch/1 -> Switch1/1
  Real-Imag to Complex1/1 -> Switch/3
  Real-Imag to Complex/1 -> Switch/1
  Constant4/1 -> Real-Imag to Complex2/1
  Constant5/1 -> Real-Imag to Complex2/2
  Constant2/1 -> Real-Imag to Complex1/1
  Constant3/1 -> Real-Imag to Complex1/2
  Constant/1 -> Real-Imag to Complex/1
  Constant1/1 -> Real-Imag to Complex/2

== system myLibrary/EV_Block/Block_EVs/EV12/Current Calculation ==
  Vp : Inport
  Constant : Constant  Commented=on  Value=2060
  Constant1 : Constant  Commented=on  Value=600
  Demux : Demux  Outputs=2
  Divide : Product  Inputs=*/
  From Workspace : FromWorkspace  VariableName=Load_Profile  SampleTime=0  OutputAfterFinalValue=Holding final value
  Gain : Gain  Gain=2
  Math Function : Math  Operator=conj
  Real-Imag to Complex : RealImagToComplex
  Isignal : Outport  VectorParamsAs1DForOutWhenUnconnected=off
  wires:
  Demux/2 -> Real-Imag to Complex/2
  Demux/1 -> Real-Imag to Complex/1
  Math Function/1 -> Isignal/1
  Divide/1 -> Math Function/1
  Gain/1 -> Divide/1
  Vp/1 -> Divide/2
  Real-Imag to Complex/1 -> Gain/1
  From Workspace/1 -> Demux/1

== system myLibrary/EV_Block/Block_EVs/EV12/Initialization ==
  Constant : Constant  Value=207.85
  Constant1 : Constant  Value=-120
  Constant2 : Constant  Value=-207.85
  Constant3 : Constant  Value=-120
  Constant4 : Constant  Value=0
  Constant5 : Constant  Value=240
  Constant6 : Constant  Value=Phase
  Data Type Conversion : DataTypeConversion  OutDataTypeStr=double
  Demux : Demux  Outputs=2
  If : If  IfExpression=u1 == 1  ElseIfExpressions=u1 == 2
  If Action Subsystem : Subsystem  TreatAsAtomicUnit=on
  If Action Subsystem1 : Subsystem  TreatAsAtomicUnit=on
  If Action Subsystem2 : Subsystem  TreatAsAtomicUnit=on
  Logical Operator : Logic  Operator=NOT  AllPortsSameDT=off  OutDataTypeStr=boolean
  Mux : Mux  Inputs=2
  Real-Imag to Complex : RealImagToComplex
  Real-Imag to Complex1 : RealImagToComplex
  Real-Imag to Complex2 : RealImagToComplex
  Switch : Switch  Criteria=u2 > Threshold
  Switch1 : Switch  Criteria=u2 > Threshold
  Out1 : Outport  VectorParamsAs1DForOutWhenUnconnected=off
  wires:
  Data Type Conversion/1 -> Mux/2
  [control] -> Demux/1
  Logical Operator/1 -> Data Type Conversion/1
  If Action Subsystem/1(Out1) -> Mux/1
  Mux/1 -> [control]
  If Action Subsystem2/1(Out1) -> Logical Operator/1
  Demux/2 -> Switch1/2
  Demux/1 -> Switch/2
  If/3 -> If Action Subsystem2/Action
  If/2 -> If Action Subsystem1/Action
  If/1 -> If Action Subsystem/Action
  Constant6/1 -> If/1
  Switch1/1 -> Out1/1
  Real-Imag to Complex2/1 -> Switch1/3
  Switch/1 -> Switch1/1
  Real-Imag to Complex1/1 -> Switch/3
  Real-Imag to Complex/1 -> Switch/1
  Constant4/1 -> Real-Imag to Complex2/1
  Constant5/1 -> Real-Imag to Complex2/2
  Constant2/1 -> Real-Imag to Complex1/1
  Constant3/1 -> Real-Imag to Complex1/2
  Constant/1 -> Real-Imag to Complex/1
  Constant1/1 -> Real-Imag to Complex/2

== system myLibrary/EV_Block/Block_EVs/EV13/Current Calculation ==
  Vp : Inport
  Constant : Constant  Commented=on  Value=2060
  Constant1 : Constant  Commented=on  Value=600
  Demux : Demux  Outputs=2
  Divide : Product  Inputs=*/
  From Workspace : FromWorkspace  VariableName=Load_Profile  SampleTime=0  OutputAfterFinalValue=Holding final value
  Gain : Gain  Gain=2
  Math Function : Math  Operator=conj
  Real-Imag to Complex : RealImagToComplex
  Isignal : Outport  VectorParamsAs1DForOutWhenUnconnected=off
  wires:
  Demux/2 -> Real-Imag to Complex/2
  Demux/1 -> Real-Imag to Complex/1
  Math Function/1 -> Isignal/1
  Divide/1 -> Math Function/1
  Gain/1 -> Divide/1
  Vp/1 -> Divide/2
  Real-Imag to Complex/1 -> Gain/1
  From Workspace/1 -> Demux/1

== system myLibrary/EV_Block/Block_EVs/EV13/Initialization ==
  Constant : Constant  Value=207.85
  Constant1 : Constant  Value=-120
  Constant2 : Constant  Value=-207.85
  Constant3 : Constant  Value=-120
  Constant4 : Constant  Value=0
  Constant5 : Constant  Value=240
  Constant6 : Constant  Value=Phase
  Data Type Conversion : DataTypeConversion  OutDataTypeStr=double
  Demux : Demux  Outputs=2
  If : If  IfExpression=u1 == 1  ElseIfExpressions=u1 == 2
  If Action Subsystem : Subsystem  TreatAsAtomicUnit=on
  If Action Subsystem1 : Subsystem  TreatAsAtomicUnit=on
  If Action Subsystem2 : Subsystem  TreatAsAtomicUnit=on
  Logical Operator : Logic  Operator=NOT  AllPortsSameDT=off  OutDataTypeStr=boolean
  Mux : Mux  Inputs=2
  Real-Imag to Complex : RealImagToComplex
  Real-Imag to Complex1 : RealImagToComplex
  Real-Imag to Complex2 : RealImagToComplex
  Switch : Switch  Criteria=u2 > Threshold
  Switch1 : Switch  Criteria=u2 > Threshold
  Out1 : Outport  VectorParamsAs1DForOutWhenUnconnected=off
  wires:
  Data Type Conversion/1 -> Mux/2
  [control] -> Demux/1
  Logical Operator/1 -> Data Type Conversion/1
  If Action Subsystem/1(Out1) -> Mux/1
  Mux/1 -> [control]
  If Action Subsystem2/1(Out1) -> Logical Operator/1
  Demux/2 -> Switch1/2
  Demux/1 -> Switch/2
  If/3 -> If Action Subsystem2/Action
  If/2 -> If Action Subsystem1/Action
  If/1 -> If Action Subsystem/Action
  Constant6/1 -> If/1
  Switch1/1 -> Out1/1
  Real-Imag to Complex2/1 -> Switch1/3
  Switch/1 -> Switch1/1
  Real-Imag to Complex1/1 -> Switch/3
  Real-Imag to Complex/1 -> Switch/1
  Constant4/1 -> Real-Imag to Complex2/1
  Constant5/1 -> Real-Imag to Complex2/2
  Constant2/1 -> Real-Imag to Complex1/1
  Constant3/1 -> Real-Imag to Complex1/2
  Constant/1 -> Real-Imag to Complex/1
  Constant1/1 -> Real-Imag to Complex/2

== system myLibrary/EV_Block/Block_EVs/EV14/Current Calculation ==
  Vp : Inport
  Constant : Constant  Commented=on  Value=2060
  Constant1 : Constant  Commented=on  Value=600
  Demux : Demux  Outputs=2
  Divide : Product  Inputs=*/
  From Workspace : FromWorkspace  VariableName=Load_Profile  SampleTime=0  OutputAfterFinalValue=Holding final value
  Gain : Gain  Gain=2
  Math Function : Math  Operator=conj
  Real-Imag to Complex : RealImagToComplex
  Isignal : Outport  VectorParamsAs1DForOutWhenUnconnected=off
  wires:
  Demux/2 -> Real-Imag to Complex/2
  Demux/1 -> Real-Imag to Complex/1
  Math Function/1 -> Isignal/1
  Divide/1 -> Math Function/1
  Gain/1 -> Divide/1
  Vp/1 -> Divide/2
  Real-Imag to Complex/1 -> Gain/1
  From Workspace/1 -> Demux/1

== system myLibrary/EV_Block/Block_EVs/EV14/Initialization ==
  Constant : Constant  Value=207.85
  Constant1 : Constant  Value=-120
  Constant2 : Constant  Value=-207.85
  Constant3 : Constant  Value=-120
  Constant4 : Constant  Value=0
  Constant5 : Constant  Value=240
  Constant6 : Constant  Value=Phase
  Data Type Conversion : DataTypeConversion  OutDataTypeStr=double
  Demux : Demux  Outputs=2
  If : If  IfExpression=u1 == 1  ElseIfExpressions=u1 == 2
  If Action Subsystem : Subsystem  TreatAsAtomicUnit=on
  If Action Subsystem1 : Subsystem  TreatAsAtomicUnit=on
  If Action Subsystem2 : Subsystem  TreatAsAtomicUnit=on
  Logical Operator : Logic  Operator=NOT  AllPortsSameDT=off  OutDataTypeStr=boolean
  Mux : Mux  Inputs=2
  Real-Imag to Complex : RealImagToComplex
  Real-Imag to Complex1 : RealImagToComplex
  Real-Imag to Complex2 : RealImagToComplex
  Switch : Switch  Criteria=u2 > Threshold
  Switch1 : Switch  Criteria=u2 > Threshold
  Out1 : Outport  VectorParamsAs1DForOutWhenUnconnected=off
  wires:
  Data Type Conversion/1 -> Mux/2
  [control] -> Demux/1
  Logical Operator/1 -> Data Type Conversion/1
  If Action Subsystem/1(Out1) -> Mux/1
  Mux/1 -> [control]
  If Action Subsystem2/1(Out1) -> Logical Operator/1
  Demux/2 -> Switch1/2
  Demux/1 -> Switch/2
  If/3 -> If Action Subsystem2/Action
  If/2 -> If Action Subsystem1/Action
  If/1 -> If Action Subsystem/Action
  Constant6/1 -> If/1
  Switch1/1 -> Out1/1
  Real-Imag to Complex2/1 -> Switch1/3
  Switch/1 -> Switch1/1
  Real-Imag to Complex1/1 -> Switch/3
  Real-Imag to Complex/1 -> Switch/1
  Constant4/1 -> Real-Imag to Complex2/1
  Constant5/1 -> Real-Imag to Complex2/2
  Constant2/1 -> Real-Imag to Complex1/1
  Constant3/1 -> Real-Imag to Complex1/2
  Constant/1 -> Real-Imag to Complex/1
  Constant1/1 -> Real-Imag to Complex/2

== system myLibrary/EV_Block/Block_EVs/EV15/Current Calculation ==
  Vp : Inport
  Constant : Constant  Commented=on  Value=2060
  Constant1 : Constant  Commented=on  Value=600
  Demux : Demux  Outputs=2
  Divide : Product  Inputs=*/
  From Workspace : FromWorkspace  VariableName=Load_Profile  SampleTime=0  OutputAfterFinalValue=Holding final value
  Gain : Gain  Gain=2
  Math Function : Math  Operator=conj
  Real-Imag to Complex : RealImagToComplex
  Isignal : Outport  VectorParamsAs1DForOutWhenUnconnected=off
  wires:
  Demux/2 -> Real-Imag to Complex/2
  Demux/1 -> Real-Imag to Complex/1
  Math Function/1 -> Isignal/1
  Divide/1 -> Math Function/1
  Gain/1 -> Divide/1
  Vp/1 -> Divide/2
  Real-Imag to Complex/1 -> Gain/1
  From Workspace/1 -> Demux/1

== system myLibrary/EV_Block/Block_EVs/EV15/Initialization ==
  Constant : Constant  Value=207.85
  Constant1 : Constant  Value=-120
  Constant2 : Constant  Value=-207.85
  Constant3 : Constant  Value=-120
  Constant4 : Constant  Value=0
  Constant5 : Constant  Value=240
  Constant6 : Constant  Value=Phase
  Data Type Conversion : DataTypeConversion  OutDataTypeStr=double
  Demux : Demux  Outputs=2
  If : If  IfExpression=u1 == 1  ElseIfExpressions=u1 == 2
  If Action Subsystem : Subsystem  TreatAsAtomicUnit=on
  If Action Subsystem1 : Subsystem  TreatAsAtomicUnit=on
  If Action Subsystem2 : Subsystem  TreatAsAtomicUnit=on
  Logical Operator : Logic  Operator=NOT  AllPortsSameDT=off  OutDataTypeStr=boolean
  Mux : Mux  Inputs=2
  Real-Imag to Complex : RealImagToComplex
  Real-Imag to Complex1 : RealImagToComplex
  Real-Imag to Complex2 : RealImagToComplex
  Switch : Switch  Criteria=u2 > Threshold
  Switch1 : Switch  Criteria=u2 > Threshold
  Out1 : Outport  VectorParamsAs1DForOutWhenUnconnected=off
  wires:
  Data Type Conversion/1 -> Mux/2
  [control] -> Demux/1
  Logical Operator/1 -> Data Type Conversion/1
  If Action Subsystem/1(Out1) -> Mux/1
  Mux/1 -> [control]
  If Action Subsystem2/1(Out1) -> Logical Operator/1
  Demux/2 -> Switch1/2
  Demux/1 -> Switch/2
  If/3 -> If Action Subsystem2/Action
  If/2 -> If Action Subsystem1/Action
  If/1 -> If Action Subsystem/Action
  Constant6/1 -> If/1
  Switch1/1 -> Out1/1
  Real-Imag to Complex2/1 -> Switch1/3
  Switch/1 -> Switch1/1
  Real-Imag to Complex1/1 -> Switch/3
  Real-Imag to Complex/1 -> Switch/1
  Constant4/1 -> Real-Imag to Complex2/1
  Constant5/1 -> Real-Imag to Complex2/2
  Constant2/1 -> Real-Imag to Complex1/1
  Constant3/1 -> Real-Imag to Complex1/2
  Constant/1 -> Real-Imag to Complex/1
  Constant1/1 -> Real-Imag to Complex/2

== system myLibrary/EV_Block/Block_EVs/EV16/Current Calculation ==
  Vp : Inport
  Constant : Constant  Commented=on  Value=2060
  Constant1 : Constant  Commented=on  Value=600
  Demux : Demux  Outputs=2
  Divide : Product  Inputs=*/
  From Workspace : FromWorkspace  VariableName=Load_Profile  SampleTime=0  OutputAfterFinalValue=Holding final value
  Gain : Gain  Gain=2
  Math Function : Math  Operator=conj
  Real-Imag to Complex : RealImagToComplex
  Isignal : Outport  VectorParamsAs1DForOutWhenUnconnected=off
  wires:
  Demux/2 -> Real-Imag to Complex/2
  Demux/1 -> Real-Imag to Complex/1
  Math Function/1 -> Isignal/1
  Divide/1 -> Math Function/1
  Gain/1 -> Divide/1
  Vp/1 -> Divide/2
  Real-Imag to Complex/1 -> Gain/1
  From Workspace/1 -> Demux/1

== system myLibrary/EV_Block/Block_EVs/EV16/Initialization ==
  Constant : Constant  Value=207.85
  Constant1 : Constant  Value=-120
  Constant2 : Constant  Value=-207.85
  Constant3 : Constant  Value=-120
  Constant4 : Constant  Value=0
  Constant5 : Constant  Value=240
  Constant6 : Constant  Value=Phase
  Data Type Conversion : DataTypeConversion  OutDataTypeStr=double
  Demux : Demux  Outputs=2
  If : If  IfExpression=u1 == 1  ElseIfExpressions=u1 == 2
  If Action Subsystem : Subsystem  TreatAsAtomicUnit=on
  If Action Subsystem1 : Subsystem  TreatAsAtomicUnit=on
  If Action Subsystem2 : Subsystem  TreatAsAtomicUnit=on
  Logical Operator : Logic  Operator=NOT  AllPortsSameDT=off  OutDataTypeStr=boolean
  Mux : Mux  Inputs=2
  Real-Imag to Complex : RealImagToComplex
  Real-Imag to Complex1 : RealImagToComplex
  Real-Imag to Complex2 : RealImagToComplex
  Switch : Switch  Criteria=u2 > Threshold
  Switch1 : Switch  Criteria=u2 > Threshold
  Out1 : Outport  VectorParamsAs1DForOutWhenUnconnected=off
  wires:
  Data Type Conversion/1 -> Mux/2
  [control] -> Demux/1
  Logical Operator/1 -> Data Type Conversion/1
  If Action Subsystem/1(Out1) -> Mux/1
  Mux/1 -> [control]
  If Action Subsystem2/1(Out1) -> Logical Operator/1
  Demux/2 -> Switch1/2
  Demux/1 -> Switch/2
  If/3 -> If Action Subsystem2/Action
  If/2 -> If Action Subsystem1/Action
  If/1 -> If Action Subsystem/Action
  Constant6/1 -> If/1
  Switch1/1 -> Out1/1
  Real-Imag to Complex2/1 -> Switch1/3
  Switch/1 -> Switch1/1
  Real-Imag to Complex1/1 -> Switch/3
  Real-Imag to Complex/1 -> Switch/1
  Constant4/1 -> Real-Imag to Complex2/1
  Constant5/1 -> Real-Imag to Complex2/2
  Constant2/1 -> Real-Imag to Complex1/1
  Constant3/1 -> Real-Imag to Complex1/2
  Constant/1 -> Real-Imag to Complex/1
  Constant1/1 -> Real-Imag to Complex/2

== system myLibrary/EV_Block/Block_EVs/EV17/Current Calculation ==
  Vp : Inport
  Constant : Constant  Commented=on  Value=2060
  Constant1 : Constant  Commented=on  Value=600
  Demux : Demux  Outputs=2
  Divide : Product  Inputs=*/
  From Workspace : FromWorkspace  VariableName=Load_Profile  SampleTime=0  OutputAfterFinalValue=Holding final value
  Gain : Gain  Gain=2
  Math Function : Math  Operator=conj
  Real-Imag to Complex : RealImagToComplex
  Isignal : Outport  VectorParamsAs1DForOutWhenUnconnected=off
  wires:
  Demux/2 -> Real-Imag to Complex/2
  Demux/1 -> Real-Imag to Complex/1
  Math Function/1 -> Isignal/1
  Divide/1 -> Math Function/1
  Gain/1 -> Divide/1
  Vp/1 -> Divide/2
  Real-Imag to Complex/1 -> Gain/1
  From Workspace/1 -> Demux/1
